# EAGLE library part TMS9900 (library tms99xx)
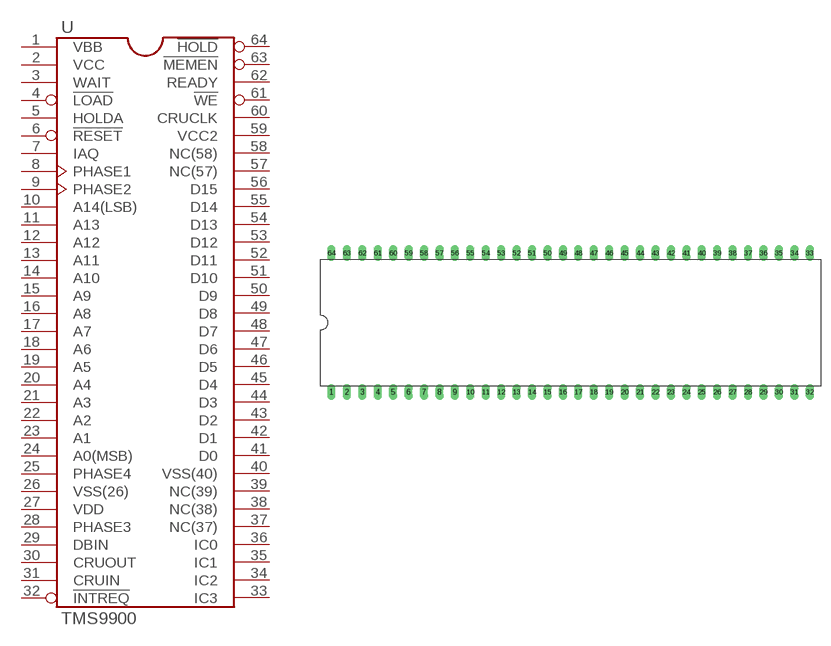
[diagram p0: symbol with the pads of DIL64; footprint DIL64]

Designator prefix -

## TMS9900  [DIL64]
1  VBB  pwr
2  VCC  pwr
3  WAIT  out
4  !LOAD  in
5  HOLDA  out
6  !RESET  in
7  IAQ  out
8  PHASE1  in
9  PHASE2  in
10  A14(LSB)  out
11  A13  out
12  A12  out
13  A11  out
14  A10  out
15  A9  out
16  A8  out
17  A7  out
18  A6  out
19  A5  out
20  A4  out
21  A3  out
22  A2  out
23  A1  out
24  A0(MSB)  out
25  PHASE4  in
26  VSS(26)  pwr
27  VDD  pwr
28  PHASE3  in
29  DBIN  out
30  CRUOUT  out
31  CRUIN  in
32  !INTREQ  in
33  IC3  in
34  IC2  in
35  IC1  in
36  IC0  in
37  NC(37)  nc
38  NC(38)  nc
39  NC(39)  nc
40  VSS(40)  pwr
41  D0
42  D1
43  D2
44  D3
45  D4
46  D5
47  D6
48  D7
49  D8
50  D9
51  D10
52  D11
53  D12
54  D13
55  D14
56  D15
57  NC(57)  nc
58  NC(58)  nc
59  VCC2  pwr
60  CRUCLK  out
61  !WE  out
62  READY  in
63  !MEMEN  out
64  !HOLD  in

## Footprint DIL64 (pad centres in mm)
drill 0.813 long: 1 -38.1,-11.43; 2 -35.56,-11.43; 3 -33.02,-11.43; 4 -30.48,-11.43; 5 -27.94,-11.43; 6 -25.4,-11.43; 7 -22.86,-11.43; 8 -20.32,-11.43; 9 -17.78,-11.43; 10 -15.24,-11.43; 11 -12.7,-11.43; 12 -10.16,-11.43; 13 -7.62,-11.43; 14 -5.08,-11.43; 15 -2.54,-11.43; 16 0,-11.43; 17 2.54,-11.43; 18 5.08,-11.43; 19 7.62,-11.43; 20 10.16,-11.43; 21 12.7,-11.43; 22 15.24,-11.43; 23 17.78,-11.43; 24 20.32,-11.43; 25 22.86,-11.43; 26 25.4,-11.43; 27 27.94,-11.43; 28 30.48,-11.43; 29 33.02,-11.43; 30 35.56,-11.43; 31 38.1,-11.43; 32 40.64,-11.43; 33 40.64,11.43; 34 38.1,11.43; 35 35.56,11.43; 36 33.02,11.43; 37 30.48,11.43; 38 27.94,11.43; 39 25.4,11.43; 40 22.86,11.43; 41 20.32,11.43; 42 17.78,11.43; 43 15.24,11.43; 44 12.7,11.43; 45 10.16,11.43; 46 7.62,11.43; 47 5.08,11.43; 48 2.54,11.43; 49 0,11.43; 50 -2.54,11.43; 51 -5.08,11.43; 52 -7.62,11.43; 53 -10.16,11.43; 54 -12.7,11.43; 55 -15.24,11.43; 56 -17.78,11.43; 57 -20.32,11.43; 58 -22.86,11.43; 59 -25.4,11.43; 60 -27.94,11.43; 61 -30.48,11.43; 62 -33.02,11.43; 63 -35.56,11.43; 64 -38.1,11.43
